(* Logix 5000 AddOnInstructionDefinition export SPEL_ResetError; software revision 30.01 *)

ADD_ON_INSTRUCTION SPEL_ResetError   (* revision 1.2 *)
// Resets AOI library error state. This AOI must be executed to clear an error.
VAR_OUTPUT
   InCycle : BOOL; {access Read Only, visible}
   Done : BOOL; {visible}
   Error : BOOL; {access Read Only, visible}
END_VAR
VAR_INPUT
   Start : BOOL; {required}
END_VAR
VAR_IN_OUT
   ExtInputs : AB:ETHERNET_MODULE_INT_128Bytes:I:0; {required}
   ExtOutputs : AB:ETHERNET_MODULE_INT_128Bytes:O:0; {required}
END_VAR
VAR_OUTPUT
   ErrCode1 : INT; {access Read Only, visible}
   ErrCode2 : INT; {access Read Only, visible}
END_VAR
VAR
   TmrReset : TIMER := (PRE := 50); {access None}
   OneShotStart : BOOL; {access None}
   OneShotStart1 : BOOL; {access None}
   StartInit : BOOL; {access None}
   TmrWaitRdy : TIMER := (PRE := 100); {access None}
END_VAR

ROUTINE Logic   (* ladder *)
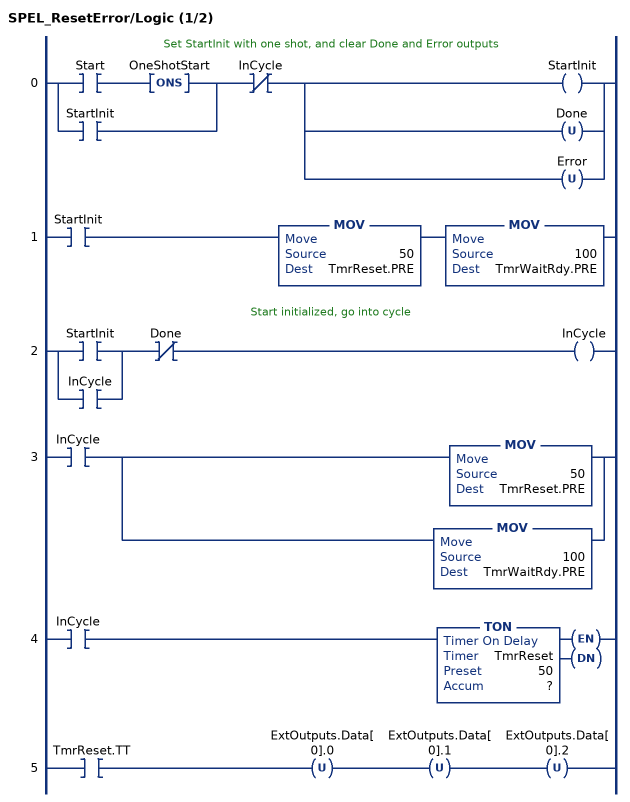
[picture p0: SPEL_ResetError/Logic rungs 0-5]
   // Set StartInit with one shot, and clear Done and Error outputs
   0: [XIC(Start) ONS(OneShotStart) ,XIC(StartInit) ]XIO(InCycle)[OTE(StartInit) ,[OTU(Done) ,OTU(Error) ] ];
   1: XIC(StartInit)MOV(50,TmrReset.PRE)MOV(100,TmrWaitRdy.PRE);
   // Start initialized, go into cycle
   2: [XIC(StartInit) ,XIC(InCycle) ]XIO(Done)OTE(InCycle);
   3: XIC(InCycle)[MOV(50,TmrReset.PRE) ,MOV(100,TmrWaitRdy.PRE) ];
   4: XIC(InCycle)TON(TmrReset,?,?);
   5: XIC(TmrReset.TT)OTU(ExtOutputs.Data[0].0)OTU(ExtOutputs.Data[0].1)OTU(ExtOutputs.Data[0].2);
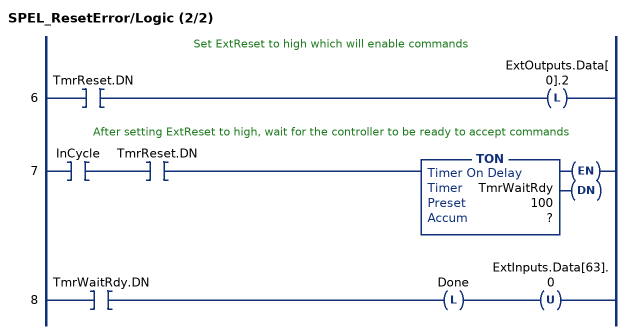
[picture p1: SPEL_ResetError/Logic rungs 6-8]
   // Set ExtReset to high which will enable commands
   6: XIC(TmrReset.DN)OTL(ExtOutputs.Data[0].2);
   // After setting ExtReset to high, wait for the controller to be ready to accept commands
   7: XIC(InCycle)XIC(TmrReset.DN)TON(TmrWaitRdy,?,?);
   8: XIC(TmrWaitRdy.DN)OTL(Done)OTU(ExtInputs.Data[63].0);
END_ROUTINE
END_ADD_ON_INSTRUCTION
